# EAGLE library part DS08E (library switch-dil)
DIL/CODE SWITCH
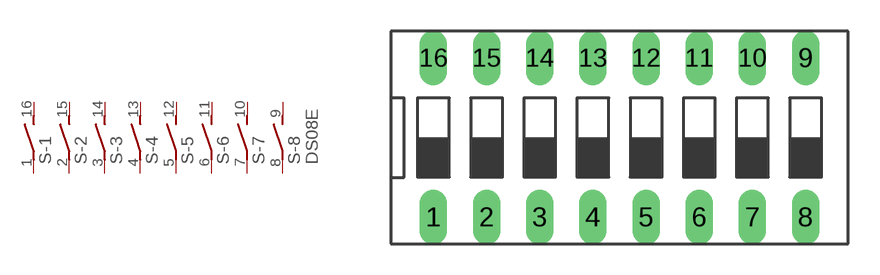
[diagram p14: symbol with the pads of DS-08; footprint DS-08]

Designator prefix S; gates -1=S -2=S -3=S -4=S -5=S -6=S -7=S -8=S+V

## DS08E (MPN: DS08; OC_FARNELL: unknown; OC_NEWARK: 73J0071)  [DS-08]
1  -1:1  pas
2  -2:1  pas
3  -3:1  pas
4  -4:1  pas
5  -5:1  pas
6  -6:1  pas
7  -7:1  pas
8  -8:1  pas
9  -8:2  pas
10  -7:2  pas
11  -6:2  pas
12  -5:2  pas
13  -4:2  pas
14  -3:2  pas
15  -2:2  pas
16  -1:2  pas

## Footprint DS-08 (pad centres in mm)
DIL/CODE SWITCH Mors distributor Buerklin, 17G562
drill 0.813 long: 1 -8.89,-3.81; 2 -6.35,-3.81; 3 -3.81,-3.81; 4 -1.27,-3.81; 5 1.27,-3.81; 6 3.81,-3.81; 7 6.35,-3.81; 8 8.89,-3.81; 9 8.89,3.81; 10 6.35,3.81; 11 3.81,3.81; 12 1.27,3.81; 13 -1.27,3.81; 14 -3.81,3.81; 15 -6.35,3.81; 16 -8.89,3.81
